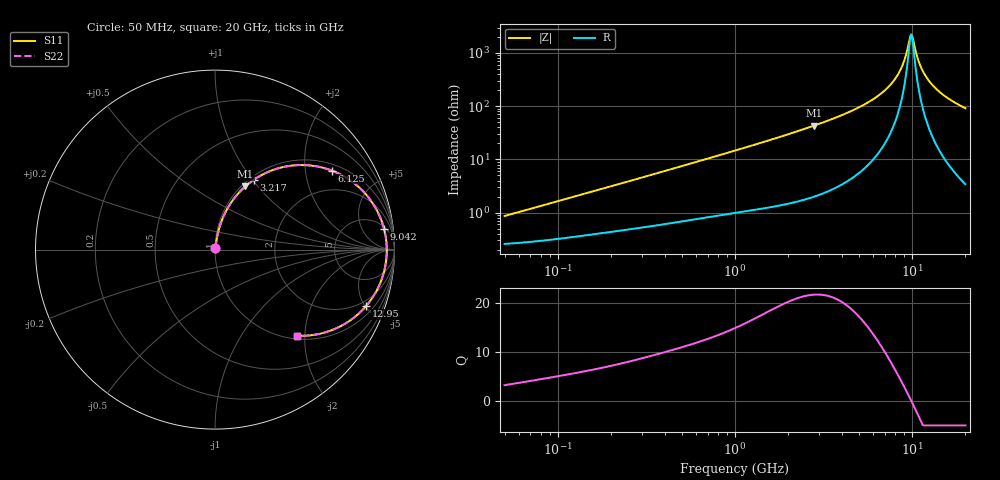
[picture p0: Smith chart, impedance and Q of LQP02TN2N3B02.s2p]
!Murata Part Number: LQP02TN2N3B02
!These Parameters are Measured in Series Mode Connection
!  o--[Z]--o
!Port1  Port2
!  o-------o
!Freq. Start=50[MHz] Stop=20[GHz], 401[Steps]
# Hz S RI R 50
!Freq.(Hz) S11(Real) S11(Imag) S21(Real) S21(Imag) S12(Real) S12(Imag) S22(Real) S22(Imag)
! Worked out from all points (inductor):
!   401 points, 50 MHz to 20 GHz, reference 50 ohm
!   read as one part in series: L = 2.61 nH near 51.52 MHz
!   highest Q = 21.6 at 2.811 GHz (marker M1), where L = 2.45 nH
!   self-resonance near 9.899 GHz
!   S11 on the Smith chart (normalised r, x): 50 MHz: 1.01, +0.02; 3.217 GHz: 1.05, +1.02; 6.125 GHz: 1.21, +2.79; 9.042 GHz: 6, +14; 12.95 GHz: 1.55, -5.08; 20 GHz: 1.07, -1.83
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5e7  0.00264 0.00821  0.9974 -0.00821  0.9974 -0.00821  0.00264 0.00821
1.364002e8  0.00411 0.0214  0.9959 -0.0214  0.9959 -0.0214  0.00411 0.0214
3.721004e8  0.00888 0.0552  0.9911 -0.0552  0.9911 -0.0552  0.00888 0.0552
1e9  0.03 0.1402  0.97 -0.1402  0.97 -0.1402  0.03 0.1402
1.793498e9  0.0762 0.2408  0.9238 -0.2408  0.9238 -0.2408  0.0762 0.2408
2.728004e9  0.1604 0.3445  0.8396 -0.3445  0.8396 -0.3445  0.1604 0.3445
2.810964e9  0.1694 0.3527  0.8306 -0.3527  0.8306 -0.3527  0.1694 0.3527
3.216634e9  0.2167 0.3894  0.7833 -0.3894  0.7833 -0.3894  0.2167 0.3894
4.748272e9  0.4352 0.4688  0.5648 -0.4688  0.5648 -0.4688  0.4352 0.4688
6.125241e9  0.6513 0.4402  0.3487 -0.4402  0.3487 -0.4402  0.6513 0.4402
7.442007e9  0.8251 0.325  0.1749 -0.325  0.1749 -0.325  0.8251 0.325
8.389408e9  0.9083 0.206  0.0917 -0.206  0.0917 -0.206  0.9083 0.206
9.041845e9  0.9416 0.1166  0.0584 -0.1166  0.0584 -0.1166  0.9416 0.1166
9.745021e9  0.9564 0.0204  0.0436 -0.0204  0.0436 -0.0204  0.9564 0.0204
9.892087e9  0.957 0.000805  0.043 -0.000805  0.043 -0.000805  0.957 0.000805
1.004137e10  0.9568 -0.0188  0.0432 0.0188  0.0432 0.0188  0.9568 -0.0188
1.082228e10  0.9437 -0.1155  0.0563 0.1155  0.0563 0.1155  0.9437 -0.1155
1.131968e10  0.9267 -0.1709  0.0733 0.1709  0.0733 0.1709  0.9267 -0.1709
1.201863e10  0.8946 -0.2396  0.1054 0.2396  0.1054 0.2396  0.8946 -0.2396
1.295331e10  0.8418 -0.3144  0.1582 0.3144  0.1582 0.3144  0.8418 -0.3144
1.550395e10  0.6829 -0.4351  0.3171 0.4351  0.3171 0.4351  0.6829 -0.4351
2e10  0.4578 -0.48  0.5422 0.48  0.5422 0.48  0.4578 -0.48
